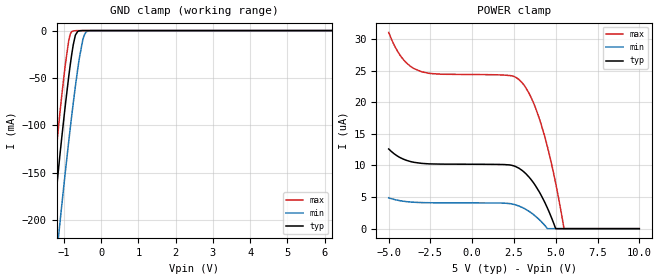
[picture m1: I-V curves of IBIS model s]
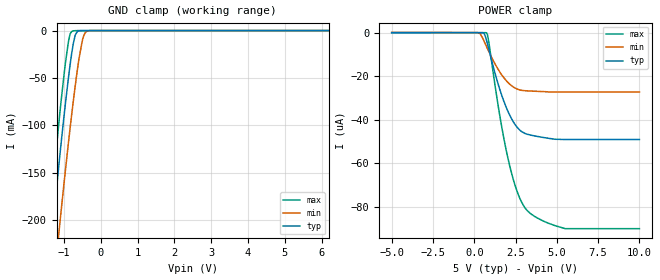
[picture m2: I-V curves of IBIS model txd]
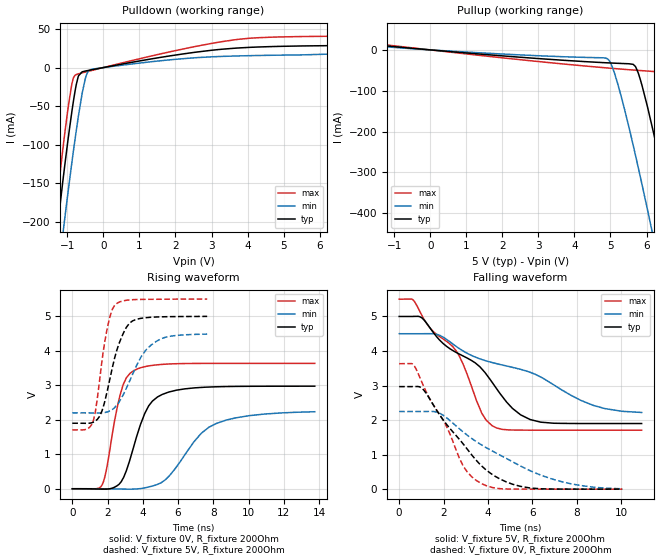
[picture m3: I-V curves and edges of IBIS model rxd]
|Texas Instruments Incorporated
|Automotive Fault Protected CAN Transceiver With Flexible Data-Rate
|Marketing part#   Digital Voltage Range   Package-type   #pins
|TCAN1051DQ1   4.5-5.5V   SOIC   8
|TCAN1051DRQ1   4.5-5.5V   SOIC   8
[IBIS Ver]   4.1
[File name]   tcan1051_q1.ibs
[File Rev]   1.0
[Date]   04/04/2016
[Source]
| Texas Instruments Incorporated.
| Analog-eLab Design Center, HPA
| 12500 TI Blvd
| Dallas, TX -75243
[Notes]   Revision History:
| Rev 1.0: 04/04/2016
| - Relative Part of TCAN1042HGV_Q1
| - Initial version of the model
| - Model generated from simulations in SPECTRE
| - Model matched to SPICE simulation
| - C_comp although listed in numerical order of value are
|   obtained from varying PVT conditions. For PVT conditions for
|   each specific value refer the buffer description under
|   respective [Model]. IBIS model user is responsible for using
|   appropriate C_comp to simulate for Signal Integrity.
|* EXCEPTION:   *
|* - For model s,there will be leakage in power clamp IV table because   *
|*   of resistor R0 connected to pad.   *
|* - For models rxd pullup and pulldown IV curves do not pass through   *
|*   zero because of resistors R6, R8, R14 connected to pad.   *
|* - For canh_os model pullup table does not pass through zero due to   *
|*   resistor network connected to PAD. Power clamp table has leakage due *
|*   to resistor network connected to PAD   *
|* - For canl_od model pulldown table does not pass through zero due to   *
|*   resistor network connected to PAD. Power clamp table has leakage due *
|*   to resistor network connected to PAD   *
[Disclaimer]
| This model is designed as an aid for customers of Texas Instruments.
| TI and its licensors and suppliers make no warranties, either expressed
| or implied, with respect to this  model, including the warranties of
| merchantability or fitness for a particular purpose. The model is
| provided solely on an "as is" basis. The entire risk as to its quality
| and performance is with the customer.
[Copyright]
(C) Copyright 2016 Texas Instruments Incorporated.All rights reserved.
|   TCAN1051_Q1D
[Component]   TCAN1051_Q1D
[Manufacturer]   TI
[Package]   |8 SOIC - D Package
|   typ   min   max
R_pkg   0.068   0.038   0.098
L_pkg   2.235nH   1.713nH   2.756nH
C_pkg   0.393pF   0.337pF   0.449pF
[Pin]  signal_name   model_name   R_pin   L_pin   C_pin
1   TXD   txd   0.093   2.653n   0.337p
2   GND   gnd   0.038   1.716n   0.449p
3   VCC   power   0.038   1.713n   0.449p
4   RXD   rxd   0.093   2.657n   0.337p
5   NC   nc   0.098   2.756n   0.341p
6   CANL   canl_od   0.092   2.624n   0.363p
7   CANH   canh_os   0.075   2.301n   0.349p
8   S   s   0.094   2.677n   0.338p
[Diff_pin]   inv_pin   vdiff   tdelay_typ   tdelay_min   tdelay_max
7   6   NA   NA   NA   NA
| Models and submodels in the file (5): s (Input), txd (Input), rxd (Output), canh_os (I/O_open_source), canl_od (I/O_open_drain)
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|   s Model
[Model]   s
Model_type   Input
Vinl = 1.5
Vinh = 3.5
|   typ   min   max
|   (nom PVT)   (fast PVT)   (slow PVT)
C_comp   2.287e-12   2.106e-12   2.744e-12
| Where nom  PVT is Nominal Process, 5V, 27C
|   Fast PVT is Strong Process,  5.5V, -55C
|   Slow PVT is Weak Process,   4.5V, 150C
[Voltage Range]   5   4.5   5.5
|Junction Temperature
[Temperature Range]   27   150   -55
[Power Clamp Reference]   5   4.5   5.5
[GND Clamp Reference]   0   0   0
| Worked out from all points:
|   GND clamp passes 1 mA (typ) near -0.63 V on its own axis
[GND Clamp]
|   Voltage   I(typ)   I(min)   I(max)
-5V       -1.891A    -1.922A    -1.879A
-1.522V   -297.1mA   -366.4mA   -255mA
-1.373V   -235.5mA   -306.2mA   -192mA
-1.115V   -133.6mA   -205.2mA   -88.92mA
-960mV    -77.4mA    -147.8mA   -34.83mA
-875mV    -49.34mA   -117.7mA   -11.3mA
-825.5mV  -34.36mA   -100.9mA   -3.168mA
-750mV    -14.77mA   -76.13mA   -399.8uA
-630mV    -843.6uA   -40.3mA    -36.57uA
-500mV    -28.97uA   -10.78mA   -9.13uA
-329mV    -2.73uA    -244.8uA   -5.367uA
10V       0A         0A         0A
[POWER Clamp]
|   Voltage   I(typ)   I(min)   I(max)
-5V       12.61uA    4.884uA    31.06uA
-4.662V   11.83uA    4.616uA    29uA
-4.114V   10.99uA    4.339uA    26.73uA
-3.031V   10.33uA    4.127uA    24.83uA
2.245V    10.08uA    3.968uA    24.23uA
2.991V    9.205uA    3.354uA    23.08uA
3.635V    7.376uA    2.292uA    20.11uA
4.297V    4.405uA    654.3nA    14.98uA
4.495V    3.293uA    0A         13.02uA
4.995V    0A         0A         7.184uA
5.494V    0A         0A         0A
10V       0A         0A         0A
|   txd Model
[Model]   txd
Model_type   Input
Vinl = 1.5
Vinh = 3.5
|   typ   min   max
|   (nom PVT)   (fast PVT)   (slow PVT)
C_comp   2.287e-12   2.118e-12   2.744e-12
| Where nom  PVT is Nominal Process, 5V, 27C
|   Fast PVT is Strong Process,  5.5V, -55C
|   Slow PVT is Weak Process,   4.5V, 150C
[Voltage Range]   5   4.5   5.5
|Junction Temperature
[Temperature Range]   27   150   -55
[Power Clamp Reference]   5   4.5   5.5
[GND Clamp Reference]   0   0   0
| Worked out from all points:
|   GND clamp passes 1 mA (typ) near -0.63 V on its own axis
[GND Clamp]
|   Voltage   I(typ)   I(min)   I(max)
-5V       -1.891A    -1.922A    -1.879A
-1.522V   -297.1mA   -366.4mA   -254.9mA
-1.373V   -235.5mA   -306.1mA   -191.9mA
-1.115V   -133.5mA   -205.2mA   -88.84mA
-960mV    -77.35mA   -147.7mA   -34.78mA
-875mV    -49.3mA    -117.7mA   -11.26mA
-825.5mV  -34.32mA   -100.8mA   -3.135mA
-750mV    -14.75mA   -76.11mA   -374.7uA
-630mV    -834.4uA   -40.28mA   -23.45uA
-500mV    -25.05uA   -10.77mA   -1.409uA
-329mV    -545.1nA   -243.3uA   -638.6nA
10V       0A         0A         0A
[POWER Clamp]
|   Voltage   I(typ)   I(min)   I(max)
-5V       0A         120.9nA    0A
211mV     0A         33.05nA    0A
560mV     -118.4nA   -3.349uA   0A
753mV     -3.857uA   -6.574uA   -165.8nA
890.5mV   -7.965uA   -8.838uA   -4.838uA
1.6V      -27.33uA   -18.67uA   -40.53uA
2.018V    -35.76uA   -22.68uA   -56.9uA
2.502V    -42.48uA   -25.54uA   -70.81uA
3.1V      -46.34uA   -26.65uA   -80.68uA
4.053V    -47.93uA   -27uA      -85.97uA
5.505V    -49.02uA   -27.21uA   -89.93uA
10V       -49.02uA   -27.21uA   -89.93uA
|   rxd Model
[Model]   rxd
Model_type   Output
Polarity   Non-Inverting
Vmeas = 2.5
Vref = 0
Cref = 2pF
Rref = 250
|   typ   min   max
|   (nom PVT)   (fast PVT)   (slow PVT)
C_comp   2.386e-12   2.168e-12   2.894e-12
| Where nom  PVT is Nominal Process, 5V, 27C
|   Fast PVT is Strong Process,  5.5V, -55C
|   Slow PVT is Weak Process,   4.5V, 150C
[Voltage Range]   5   4.5   5.5
|Junction Temperature
[Temperature Range]   27   150   -55
[Pullup Reference]   5   4.5   5.5
[Pulldown Reference]   0   0   0
[Power Clamp Reference]   5   4.5   5.5
[GND Clamp Reference]   0   0   0
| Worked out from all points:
|   slope of the pulldown table from 0 to 0.75 V, typ, clamps not added: 115 ohm
|   slope of the pullup table from 0 to 0.75 V, typ, clamps not added: 132 ohm
|   falling waveform, V_fixture 5V, R_fixture 200Ohm: 20-80 % time 3.11ns typ, 5.09ns min, 2.25ns max; typ from 5 V to 1.9 V
|   rising waveform, V_fixture 0V, R_fixture 200Ohm: 20-80 % time 1.2ns typ, 2.14ns min, 823ps max; typ from 0 V to 2.97 V
|   rising waveform, V_fixture 5V, R_fixture 200Ohm: 20-80 % time 946ps typ, 1.37ns min, 646ps max; typ from 1.9 V to 5 V
|   falling waveform, V_fixture 0V, R_fixture 200Ohm: 20-80 % time 2.25ns typ, 3.56ns min, 1.68ns max; typ from 2.97 V to 0.001 V
[Pulldown]
|   Voltage   I(typ)   I(min)   I(max)
-5V       -1.938A    -1.963A    -1.932A
-1.377V   -248.8mA   -316mA     -209.1mA
-1.13V    -148.8mA   -217.5mA   -107.2mA
-1.073V   -127mA     -195.6mA   -85.47mA
-875mV    -56.91mA   -122.9mA   -21.26mA
-702.5mV  -12.29mA   -65.58mA   -8.197mA
-500mV    -4.424mA   -13.85mA   -5.745mA
-324.5mV  -2.846mA   -2.215mA   -3.716mA
3.728V    25.37mA    15.1mA     36.53mA
6.803V    28.7mA     18.18mA    40.78mA
8.045V    29.33mA    26.87mA    41.11mA
10V       47.12mA    41.2mA     50.1mA
[Pullup]
|   Voltage   I(typ)   I(min)   I(max)
-5V       40.48mA    32.39mA    49.71mA
4.886V    -31.59mA   -20.71mA   -44.08mA
5.115V    -32.54mA   -58.15mA   -45.76mA
5.63V     -35.43mA   -233.7mA   -49.34mA
5.818V    -69.8mA    -307.1mA   -50.55mA
6.025V    -138.9mA   -390.8mA   -51.84mA
6.191V    -202mA     -459.7mA   -52.94mA
6.357V    -268.5mA   -529.6mA   -63.55mA
6.72V     -421.4mA   -685.5mA   -189.1mA
7.105V    -590.7mA   -855.6mA   -352.4mA
7.405V    -725.6mA   -991.5mA   -486.5mA
10V       -1.941A    -2.202A    -1.705A
[Ramp]
R_load = 200
|   typ   min   max
dV/dt_r   1.78423/1.19645e-09   1.35379/2.20652e-09   2.1811/8.22747e-10
dV/dt_f   1.86055/3.10845e-09   1.38029/5.12898e-09   2.27576/2.25078e-09
[Falling Waveform]
V_fixture = 5V
V_fixture_min = 4.5V
V_fixture_max = 5.5V
R_fixture = 200Ohm
|   Time   V(typ)   V(min)   V(max)
0s        5V         4.5V       5.5V
597.3ps   5.001V     4.5V       5.494V
1.021ns   4.959V     4.5V       5.033V
2.562ns   3.961V     4.136V     4.01V
3.717ns   3.485V     3.756V     2.204V
4.187ns   3.093V     3.666V     1.837V
5.102ns   2.338V     3.527V     1.713V
5.898ns   2.016V     3.384V     1.709V
8.726ns   1.9V       2.429V     1.708V
10.92ns   1.9V       2.221V     1.707V
[Rising Waveform]
V_fixture = 0V
V_fixture_min = 0V
V_fixture_max = 0V
R_fixture = 200Ohm
|   Time   V(typ)   V(min)   V(max)
0s        83.56pV    37.66nV    52.85pV
1.696ns   -11.4mV    -764.2uV   113.6mV
1.945ns   -10.34mV   -2.302mV   569mV
2.708ns   162.5mV    -8.668mV   2.71V
3.474ns   1.198V     -10.36mV   3.419V
4.337ns   2.405V     51.96mV    3.561V
5.472ns   2.803V     358.2mV    3.617V
7.316ns   2.937V     1.606V     3.634V
8.161ns   2.956V     1.89V      3.635V
13.76ns   2.973V     2.232V     3.635V
[Rising Waveform]
V_fixture = 5V
V_fixture_min = 4.5V
V_fixture_max = 5.5V
R_fixture = 200Ohm
|   Time   V(typ)   V(min)   V(max)
0s        1.899V     2.2V       1.707V
871.2ps   1.897V     2.199V     1.742V
1.21ns    1.933V     2.197V     1.999V
1.551ns   2.101V     2.196V     3.146V
1.945ns   2.746V     2.222V     4.548V
2.407ns   3.799V     2.355V     5.319V
3.243ns   4.798V     3.11V      5.475V
4.469ns   4.972V     4.164V     5.492V
5.531ns   4.989V     4.42V      5.496V
7.654ns   4.997V     4.484V     5.5V
[Falling Waveform]
V_fixture = 0V
V_fixture_min = 0V
V_fixture_max = 0V
R_fixture = 200Ohm
|   Time   V(typ)   V(min)   V(max)
0s        2.969V     2.248V     3.633V
597.3ps   2.97V      2.248V     3.626V
1.021ns   2.925V     2.249V     3.099V
1.854ns   2.122V     2.19V      2.131V
2.884ns   1.309V     1.655V     668.9mV
3.717ns   672.3mV    1.28V      159mV
4.836ns   207.1mV    887.3mV    5.685mV
5.898ns   34.39mV    535.8mV    1.224mV
7.747ns   1.562mV    154.6mV    636.8uV
10.04ns   719.3uV    10.71mV    385.9uV
